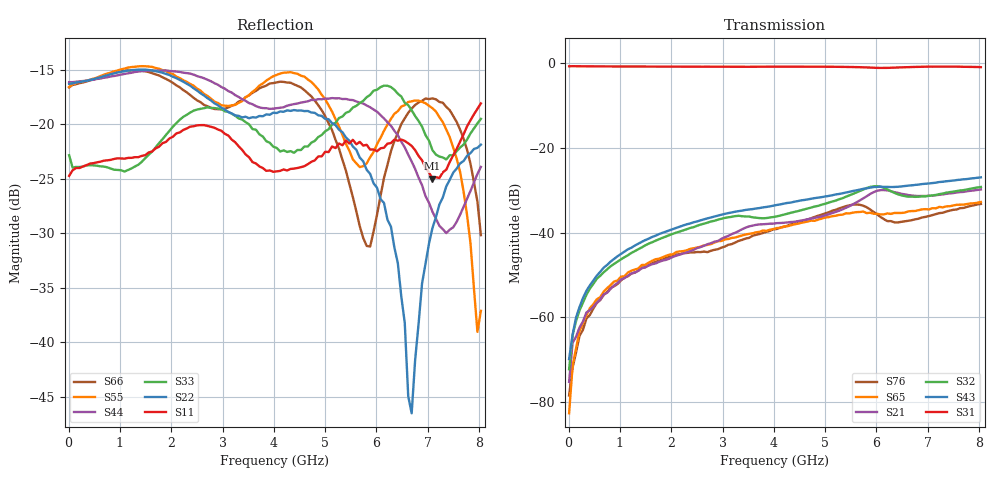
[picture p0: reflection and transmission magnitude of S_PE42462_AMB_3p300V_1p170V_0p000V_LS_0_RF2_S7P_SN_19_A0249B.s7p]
! Device ID: PE42462
! File Path: z:\PE42462\DataSheet S-parameter-6T\AMB\3p300\LS_0_RF2\PE42462_AMB_3p300V_1p170V_0p000V_LS_0_RF2_S7P_SN_19_A0249B.s7p
! Serial: 19
! Lot: A0249B
! Temp: AMB
! VDD: 3.300
! VSS: 0.000
! Control_Hi: 1.170
! Control_Lo: 0.000
! Logic State: LS_0_RF2
! Port 1:
! Port 2:
! Port 3:
! Port 4:
! Port 5:
! Port 6:
! Port 7:
! ThroughPath:1-3
! IDD: 0.0001058755
! ISS/IDD2: -1.67e-008
! IDMM3/IDD3: -2.256e-007
! Comment:
#  Hz  S  RI  R  50
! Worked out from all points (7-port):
!   120 points, 10 MHz to 8.037 GHz, reference 50 ohm
!   strongest paths, dB at 10 MHz, 2.034 GHz, 4.057 GHz, 6.08 GHz, 8.037 GHz:
!     S31: -0.8, -0.9, -0.9, -1.2, -1.0
!     S43: -69.9, -39.2, -33.5, -29.2, -27.0
!     S32: -72.2, -40.3, -36.2, -29.2, -29.3
!     S21: -75.2, -45.7, -37.8, -30.0, -29.8
!     S65: -82.6, -45.1, -38.9, -35.7, -32.8
!     S76: -78.4, -45.5, -39.2, -36.3, -33.3
!   lowest |S11| = -25.0 dB at 7.092 GHz (marker M1), VSWR 1.12, Z = 55.1 + j2.98 ohm
!   |S11| at or under -10 dB: start of sweep to end of sweep
